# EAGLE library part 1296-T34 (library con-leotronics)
1.27mm SINGLE ROW FEMALE SOCKET Source: http://www.leotronics.co.uk/Conexcon/Data%20Sheets/sec.%20A/1296ing.pdf
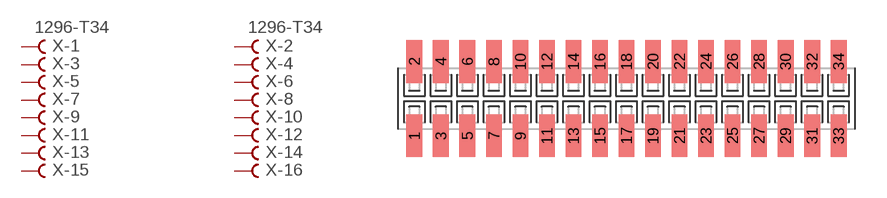
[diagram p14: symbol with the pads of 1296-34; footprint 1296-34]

Designator prefix X; gates -1=FVAL -2=FVAL -3=F -4=F -5=F -6=F -7=F -8=F -9=F -10=F -11=F -12=F -13=F -14=F -15=F -16=F -17=F -18=F -19=F -20=F -21=F -22=F -23=F -24=F -25=F -26=F -27=F -28=F -29=F -30=F -31=F -32=F -33=F -34=F

## 1296-T34 (OC_FARNELL: unknown; OC_NEWARK: unknown)  [1296-34]
1  -1:B  pas
2  -2:B  pas
3  -3:B  pas
4  -4:B  pas
5  -5:B  pas
6  -6:B  pas
7  -7:B  pas
8  -8:B  pas
9  -9:B  pas
10  -10:B  pas
11  -11:B  pas
12  -12:B  pas
13  -13:B  pas
14  -14:B  pas
15  -15:B  pas
16  -16:B  pas
17  -17:B  pas
18  -18:B  pas
19  -19:B  pas
20  -20:B  pas
21  -21:B  pas
22  -22:B  pas
23  -23:B  pas
24  -24:B  pas
25  -25:B  pas
26  -26:B  pas
27  -27:B  pas
28  -28:B  pas
29  -29:B  pas
30  -30:B  pas
31  -31:B  pas
32  -32:B  pas
33  -33:B  pas
34  -34:B  pas

## Footprint 1296-34 (pad centres in mm)
1.27mm SINGLE ROW FEMALE SOCKET Source: http://www.leotronics.co.uk/Conexcon/Data%20Sheets/sec.%20A/1296ing.pdf
smd 0.76 x 2.05: 1 -10.16,-1.78; 2 -10.16,1.78; 3 -8.89,-1.78; 4 -8.89,1.78; 5 -7.62,-1.78; 6 -7.62,1.78; 7 -6.35,-1.78; 8 -6.35,1.78; 9 -5.08,-1.78; 10 -5.08,1.78; 11 -3.81,-1.78; 12 -3.81,1.78; 13 -2.54,-1.78; 14 -2.54,1.78; 15 -1.27,-1.78; 16 -1.27,1.78; 17 0,-1.78; 18 0,1.78; 19 1.27,-1.78; 20 1.27,1.78; 21 2.54,-1.78; 22 2.54,1.78; 23 3.81,-1.78; 24 3.81,1.78; 25 5.08,-1.78; 26 5.08,1.78; 27 6.35,-1.78; 28 6.35,1.78; 29 7.62,-1.78; 30 7.62,1.78; 31 8.89,-1.78; 32 8.89,1.78; 33 10.16,-1.78; 34 10.16,1.78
